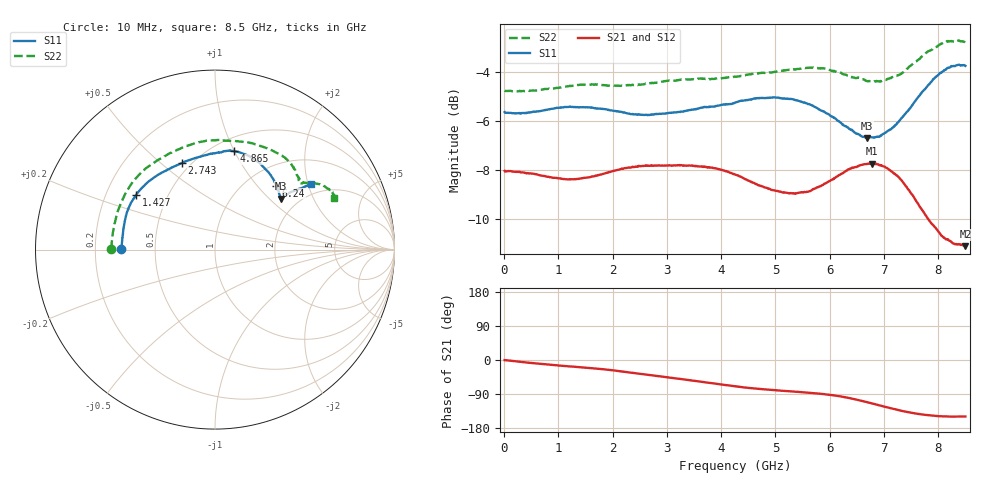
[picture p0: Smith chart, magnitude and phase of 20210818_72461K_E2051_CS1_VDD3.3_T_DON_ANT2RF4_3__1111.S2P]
!Agilent Technologies,E5071C,MY46417908,A.11.23
!Date: Wed Aug 18 14:34:46 2021
!Data & Calibration Information:
!Freq	S11:SOLT2(ON)	S21:SOLT2(ON)	S12:SOLT2(ON)	S22:SOLT2(ON)
!PortZ  Port1:50+j0  Port2:50+j0
!Above PortZ is port z conversion or system Z0 setting when saving the data.
!When reading, reference impedance value at option line is always used.
# Hz S dB R 50
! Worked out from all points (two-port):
!   1601 points, 10 MHz to 8.5 GHz, reference 50 ohm
!   highest |S21| = -7.73 dB at 6.77 GHz (marker M1); lowest = -11.1 dB at 8.5 GHz (marker M2)
!   |S21| within 3 dB of the highest: start of sweep to 8.096 GHz
!   lowest |S11| = -6.7 dB at 6.691 GHz (marker M3), VSWR 2.73, Z = 81.2 + j58.9 ohm
!   |S11| at or under -10 dB: nowhere
!   |S22| runs from -4.8 to -2.7 dB; largest |S21 - S12| = 0.0015
!   S11 on the Smith chart (normalised r, x): 10 MHz: 0.31, +0.00; 1.427 GHz: 0.33, +0.28; 2.743 GHz: 0.45, +0.59; 4.865 GHz: 0.63, +1.00; 6.24 GHz: 1.35, +1.27; 8.5 GHz: 1.65, +2.09
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1e7  -5.64 179.6  -8.03 -0.3  -8.02 -0.3  -4.76 179.6
7.847125e8  -5.54 161.3  -8.26 -11.9  -8.25 -11.9  -4.70 158.5
1.108394e9  -5.43 153.4  -8.36 -15.7  -8.35 -15.8  -4.60 148.6
1.426769e9  -5.44 145.3  -8.33 -19.3  -8.33 -19.3  -4.52 139.4
2.010456e9  -5.58 130.3  -8.02 -27.2  -8.03 -27.3  -4.55 123.0
2.742719e9  -5.73 111.0  -7.81 -40.7  -7.81 -40.8  -4.46 104.8
2.843538e9  -5.71 108.9  -7.81 -42.5  -7.80 -42.6  -4.43 102.6
3.5758e9  -5.49 94.1  -7.84 -56.3  -7.83 -56.3  -4.28 88.7
4.255e9  -5.26 85.7  -8.17 -69.3  -8.17 -69.4  -4.20 78.1
4.865219e9  -5.06 78.8  -8.74 -78.3  -8.74 -78.3  -4.04 68.4
5.31625e9  -5.12 70.4  -8.94 -83.1  -8.95 -83.0  -3.91 59.5
5.671769e9  -5.36 61.8  -8.80 -86.8  -8.82 -86.8  -3.83 53.0
5.942388e9  -5.69 53.9  -8.51 -90.8  -8.53 -90.8  -3.89 48.5
6.239538e9  -6.14 46.2  -8.12 -97.1  -8.13 -97.2  -4.09 44.1
6.457094e9  -6.46 41.4  -7.88 -103.5  -7.89 -103.6  -4.24 40.6
6.690569e9  -6.68 37.9  -7.75 -111.5  -7.74 -111.5  -4.38 39.2
6.770162e9  -6.66 37.6  -7.73 -114.3  -7.74 -114.3  -4.37 38.6
7.088538e9  -6.38 37.4  -7.96 -126.1  -7.98 -126.1  -4.28 37.1
7.385688e9  -5.72 37.4  -8.59 -136.1  -8.60 -136.1  -3.95 35.8
7.826106e9  -4.52 35.4  -10.02 -145.8  -10.00 -145.9  -3.16 31.5
8.123256e9  -3.92 34.5  -10.77 -148.7  -10.75 -148.8  -2.79 27.1
8.5e9  -3.76 34.5  -11.09 -149.0  -11.07 -149.1  -2.83 23.4
